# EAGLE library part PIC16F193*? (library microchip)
Flash-Based, 8-Bit CMOS Microcontrollers wtih LCD Driver and nanoWatt XLP Technology Auto generated by make-symbol-device-package-bsdl.ulp Rev. 33 Source: http://ww1.microchip.com/downloads/en/DeviceDoc/41364D.pdf
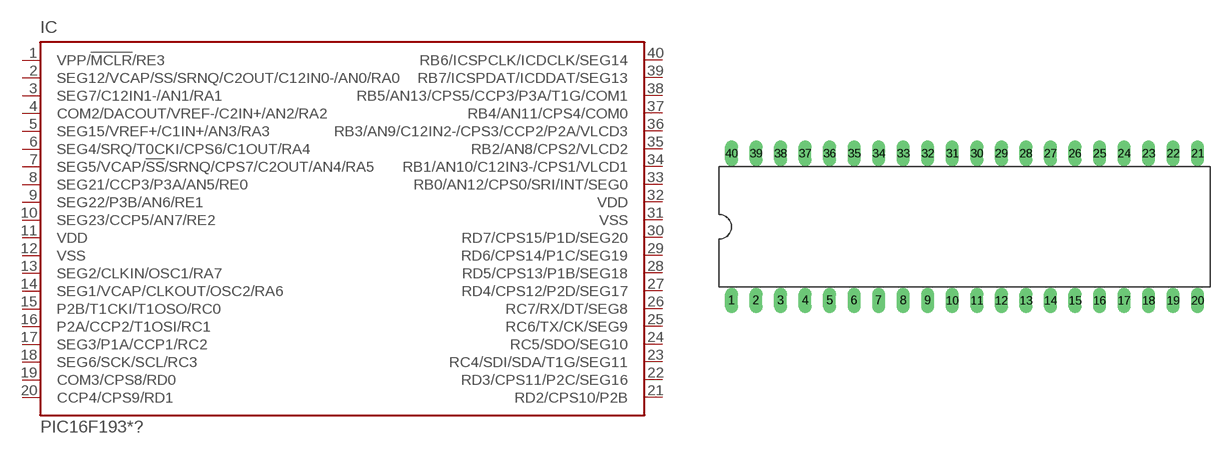
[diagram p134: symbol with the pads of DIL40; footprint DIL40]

Designator prefix IC

## PIC16F1934P (MPN: PIC16F1934-I/P; OC_FARNELL: 1755817; OC_NEWARK: 45P4755), PIC16F1937P (MPN: PIC16F1937-I/P; OC_FARNELL: 1755825; OC_NEWARK: 45P4774), PIC16F1939P (MPN: PIC16F1939-I/P; OC_FARNELL: 1755832; OC_NEWARK: 08R1958)  [DIL40]
1  VPP/!MCLR!/RE3  in
2  SEG12/VCAP/SS/SRNQ/C2OUT/C12IN0-/AN0/RA0
3  SEG7/C12IN1-/AN1/RA1
4  COM2/DACOUT/VREF-/C2IN+/AN2/RA2
5  SEG15/VREF+/C1IN+/AN3/RA3
6  SEG4/SRQ/T0CKI/CPS6/C1OUT/RA4
7  SEG5/VCAP/!SS!/SRNQ/CPS7/C2OUT/AN4/RA5
8  SEG21/CCP3/P3A/AN5/RE0
9  SEG22/P3B/AN6/RE1
10  SEG23/CCP5/AN7/RE2
11  VDD  pwr
12  VSS  pwr
13  SEG2/CLKIN/OSC1/RA7
14  SEG1/VCAP/CLKOUT/OSC2/RA6
15  P2B/T1CKI/T1OSO/RC0
16  P2A/CCP2/T1OSI/RC1
17  SEG3/P1A/CCP1/RC2
18  SEG6/SCK/SCL/RC3
19  COM3/CPS8/RD0
20  CCP4/CPS9/RD1
21  RD2/CPS10/P2B
22  RD3/CPS11/P2C/SEG16
23  RC4/SDI/SDA/T1G/SEG11
24  RC5/SDO/SEG10
25  RC6/TX/CK/SEG9
26  RC7/RX/DT/SEG8
27  RD4/CPS12/P2D/SEG17
28  RD5/CPS13/P1B/SEG18
29  RD6/CPS14/P1C/SEG19
30  RD7/CPS15/P1D/SEG20
31  VSS  pwr
32  VDD  pwr
33  RB0/AN12/CPS0/SRI/INT/SEG0
34  RB1/AN10/C12IN3-/CPS1/VLCD1
35  RB2/AN8/CPS2/VLCD2
36  RB3/AN9/C12IN2-/CPS3/CCP2/P2A/VLCD3
37  RB4/AN11/CPS4/COM0
38  RB5/AN13/CPS5/CCP3/P3A/T1G/COM1
39  RB7/ICSPDAT/ICDDAT/SEG13
40  RB6/ICSPCLK/ICDCLK/SEG14

## Footprint DIL40 (pad centres in mm)
Dual In Line package type P
drill 0.813 long: 1 -24.13,-7.62; 2 -21.59,-7.62; 3 -19.05,-7.62; 4 -16.51,-7.62; 5 -13.97,-7.62; 6 -11.43,-7.62; 7 -8.89,-7.62; 8 -6.35,-7.62; 9 -3.81,-7.62; 10 -1.27,-7.62; 11 1.27,-7.62; 12 3.81,-7.62; 13 6.35,-7.62; 14 8.89,-7.62; 15 11.43,-7.62; 16 13.97,-7.62; 17 16.51,-7.62; 18 19.05,-7.62; 19 21.59,-7.62; 20 24.13,-7.62; 21 24.13,7.62; 22 21.59,7.62; 23 19.05,7.62; 24 16.51,7.62; 25 13.97,7.62; 26 11.43,7.62; 27 8.89,7.62; 28 6.35,7.62; 29 3.81,7.62; 30 1.27,7.62; 31 -1.27,7.62; 32 -3.81,7.62; 33 -6.35,7.62; 34 -8.89,7.62; 35 -11.43,7.62; 36 -13.97,7.62; 37 -16.51,7.62; 38 -19.05,7.62; 39 -21.59,7.62; 40 -24.13,7.62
